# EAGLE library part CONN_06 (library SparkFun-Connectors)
Multi connection point. Often used as Generic Header-pin footprint for 0.1 inch spaced/style header connections On any of the 0.1 inch spaced packages, you can populate with these: Break Away Headers - Straight (PRT-00116) Break Away Male Headers - Right Angle (PRT-00553) Female Headers (PRT-00115) Break Away Headers - Machine Pin (PRT-00117) Break Away Female Headers - Swiss Machine Pin (PRT-00743) Arduino Stackable Header - 6 Pin (PRT-09280) For SCREWTERMINALS and SPRING TERMINALS visit here: Screw Terimnals on SparkFun.com (5mm/3.5mm/2.54mm spacing) This device is also useful as a general connection point to wire up your design to another part of your project. Our various solder wires solder well into these plated through hole pads. Hook-Up Wire - Assortment (Stranded, 22 AWG) (PRT-11375) Hook-Up Wire - Assortment (Solid Core, 22 AWG) (PRT-11367) View the entire wire category on our website here
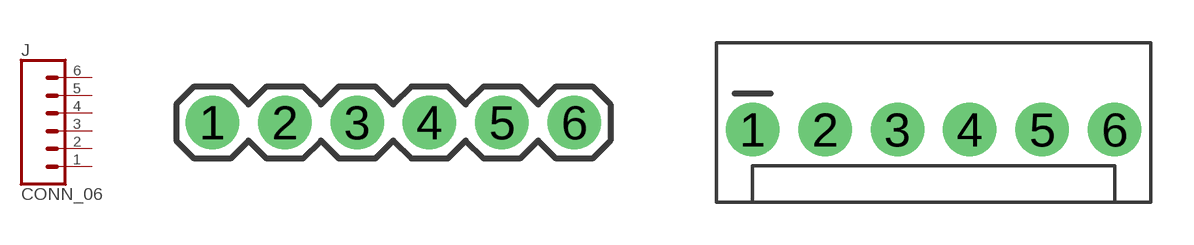
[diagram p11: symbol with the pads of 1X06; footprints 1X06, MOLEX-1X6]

Designator prefix J

## CONN_06SILK_FEMALE_PTH (PROD_ID: CONN-08437)  [1X06]
1  1  pas
2  2  pas
3  3  pas
4  4  pas
5  5  pas
6  6  pas

## CONN_06POLAR  [MOLEX-1X6]
Pads as for 1X06

## CONN_06RA  [MOLEX-1X6-RA]
Pads as for 1X06

## CONN_06SMD (PROD_ID: CONN-08971; VALUE: RA 6Pin SMD)  [1X06-SMD_RA_MALE]
Pads as for 1X06

## CONN_06LOCK  [1X06_LOCK]
Pads as for 1X06

## CONN_06LOCK_LONGPADS  [1X06_LOCK_LONGPADS]
Pads as for 1X06

## CONN_06POLAR_LOCK  [MOLEX-1X6_LOCK]
Pads as for 1X06

## CONN_06RA_LOCK  [MOLEX_1X6_RA_LOCK]
Pads as for 1X06

## CONN_06FEMALE_LOCK  [1X06_FEMALE_LOCK.010]
Pads as for 1X06

## CONN_06LONGPADS  [1X06_LONGPADS]
Pads as for 1X06

## CONN_063.5MM-6  [SCREWTERMINAL-3.5MM-6]
Pads as for 1X06

## CONN_06SMD-FEMALE-V2 (PROD_ID: CONN-09668)  [1X06-SMD-FEMALE]
Pads as for 1X06

## CONN_06POGOPIN_HOLES_ONLY (PROD_ID: CONN-08437)  [1X06_HOLES_ONLY]
Pads as for 1X06

## CONN_06SMD-STRAIGHT-FEMALE (PROD_ID: CONN-10203)  [1X06_SMD_STRAIGHT]
Pads as for 1X06

## CONN_06SMD-STRAIGHT-ALT-FEMALE (PROD_ID: CONN-10203)  [1X06_SMD_STRAIGHT_ALT]
Pads as for 1X06

## CONN_06SMD-STRAIGHT-COMBO-FEMALE (PROD_ID: CONN-10203)  [1X06_SMD_STRAIGHT_COMBO]
Pads as for 1X06

## CONN_06SMD_MALE (PROD_ID: CONN-11293)  [1X06_SMD_MALE]
Pads as for 1X06

## CONN_06SMD-1MM (PROD_ID: CONN-08249; SF_ID: GPS-00579)  [1X06-1MM]
Pads as for 1X06

## CONN_06NO_SILK_FEMALE_PTH (PROD_ID: CONN-08437)  [1X06_NO_SILK]
Pads as for 1X06

## CONN_061.27MM  [1X06_1.27MM]
Pads as for 1X06

## CONN_06NO_SILK_NO_POP  [1X06_NO_SILK]
Pads as for 1X06

## CONN_062.5MM-6-90  [1X06_SCREW_TERMINAL_BLOCK]
Pads as for 1X06

## Footprint 1X06 (pad centres in mm)
Plated Through Hole - 6 Pin Specifications: Pin count:6 Pin pitch:0.1" Example device(s): CONN_06
drill 1.016 pad 1.88: 1 0,0; 2 2.54,0; 3 5.08,0; 4 7.62,0; 5 10.16,0; 6 12.7,0

## Footprint MOLEX-1X6 (pad centres in mm)
Molex 6-Pin Plated Through-Hole Specifications: Pin count:6 Pin pitch:0.1" Datasheet referenced for footprint Example device(s): CONN_06
drill 1.016 pad 1.88: 1 0,0; 2 2.54,0; 3 5.08,0; 4 7.62,0; 5 10.16,0; 6 12.7,0

## Footprint MOLEX-1X6-RA (pad centres in mm)
Molex 6-Pin Plated Through-Hole Right Angle tPlace shows angle of connector. Specifications: Pin count:6 Pin pitch:0.1" Datasheet referenced for footprint Example device(s): CONN_06
drill 1.016 pad 1.88: 1 0,0; 2 2.54,0; 3 5.08,0; 4 7.62,0; 5 10.16,0; 6 12.7,0

## Footprint 1X06-SMD_RA_MALE (pad centres in mm)
SMD - 6 Pin Right Angle Male Header tDocu layer shows pin locations. Specifications: Pin count:6 Pin pitch:0.1" Example device(s): CONN_06
smd 1 x 3: 1 -6.35,5; 2 -3.81,5; 3 -1.27,5; 4 1.27,5; 5 3.81,5; 6 6.35,5
hole 1.4 at -5.08,0
hole 1.4 at 5.08,0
